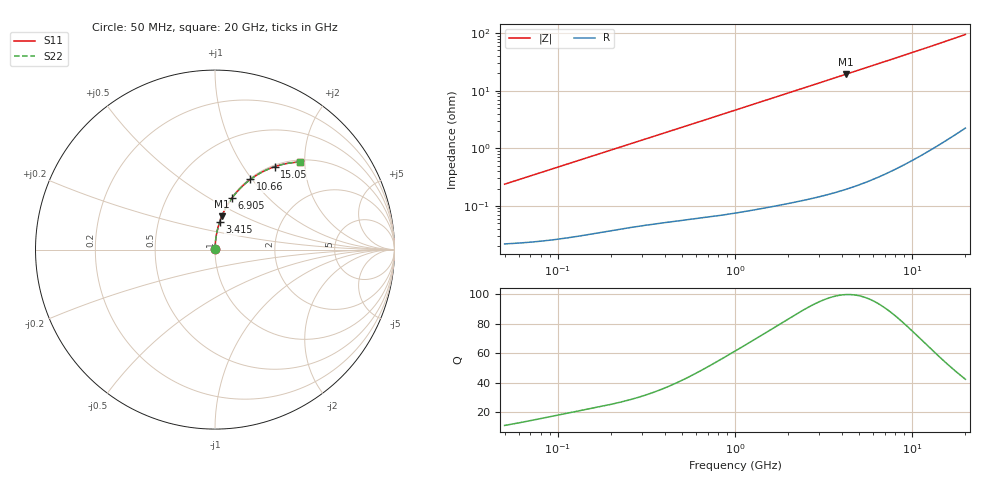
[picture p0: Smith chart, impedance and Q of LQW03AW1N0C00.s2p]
!Murata Part Number: LQW03AW1N0C00
!These Parameters are Measured in Series Mode Connection
!  o--[Z]--o
!Port1  Port2
!  o-------o
!Freq. Start=50[MHz] Stop=20[GHz], 401[Steps]
# Hz S RI R 50
!Freq.(Hz) S11(Real) S11(Imag) S21(Real) S21(Imag) S12(Real) S12(Imag) S22(Real) S22(Imag)
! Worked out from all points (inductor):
!   401 points, 50 MHz to 20 GHz, reference 50 ohm
!   read as one part in series: L = 754 pH near 51.52 MHz
!   highest Q = 99.8 at 4.212 GHz (marker M1), where L = 727 pH
!   S11 on the Smith chart (normalised r, x): 50 MHz: 1.00, +0.00; 3.415 GHz: 1.00, +0.31; 6.905 GHz: 1.01, +0.63; 10.66 GHz: 1.01, +0.98; 15.05 GHz: 1.03, +1.40; 20 GHz: 1.04, +1.90
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5e7  0.000224 0.00237  0.9998 -0.00237  0.9998 -0.00237  0.000224 0.00237
5.152053e7  0.000225 0.00244  0.9998 -0.00244  0.9998 -0.00244  0.000225 0.00244
1.364002e8  0.000345 0.00641  0.9997 -0.00641  0.9997 -0.00641  0.000345 0.00641
3.721004e8  0.000791 0.0172  0.9992 -0.0172  0.9992 -0.0172  0.000791 0.0172
6.380365e8  0.00147 0.0293  0.9985 -0.0293  0.9985 -0.0293  0.00147 0.0293
1e9  0.00284 0.0457  0.9972 -0.0457  0.9972 -0.0457  0.00284 0.0457
1.329223e9  0.00455 0.0605  0.9955 -0.0605  0.9955 -0.0605  0.00455 0.0605
1.714689e9  0.00709 0.0778  0.9929 -0.0778  0.9929 -0.0778  0.00709 0.0778
2.179053e9  0.0109 0.0984  0.9891 -0.0984  0.9891 -0.0984  0.0109 0.0984
2.728004e9  0.0166 0.1223  0.9834 -0.1223  0.9834 -0.1223  0.0166 0.1223
3.415248e9  0.0252 0.1517  0.9748 -0.1517  0.9748 -0.1517  0.0252 0.1517
4.212059e9  0.0374 0.1848  0.9626 -0.1848  0.9626 -0.1848  0.0374 0.1848
5.515528e9  0.0619 0.2358  0.9381 -0.2358  0.9381 -0.2358  0.0619 0.2358
6.905011e9  0.0934 0.2855  0.9066 -0.2855  0.9066 -0.2855  0.0934 0.2855
7.442007e9  0.1068 0.3033  0.8932 -0.3033  0.8932 -0.3033  0.1068 0.3033
8.907419e9  0.1463 0.3473  0.8537 -0.3473  0.8537 -0.3473  0.1463 0.3473
1.066139e10  0.1977 0.3913  0.8023 -0.3913  0.8023 -0.3913  0.1977 0.3913
1.257102e10  0.2561 0.4287  0.7439 -0.4287  0.7439 -0.4287  0.2561 0.4287
1.504638e10  0.3324 0.4621  0.6676 -0.4621  0.6676 -0.4621  0.3324 0.4621
1.747767e10  0.4047 0.4805  0.5953 -0.4805  0.5953 -0.4805  0.4047 0.4805
1.940974e10  0.4586 0.4869  0.5414 -0.4869  0.5414 -0.4869  0.4586 0.4869
2e10  0.4744 0.4877  0.5256 -0.4877  0.5256 -0.4877  0.4744 0.4877
